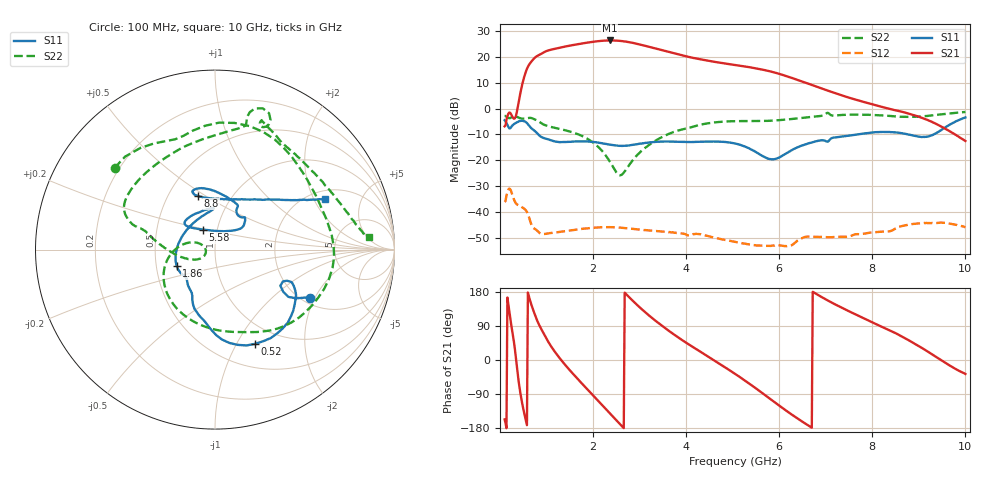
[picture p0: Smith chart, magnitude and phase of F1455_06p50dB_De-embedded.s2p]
! Integrated Device Technology
! Corporate Headquarters
! 6024 Silver Creek Valley Road
! San Jose, CA 95138  USA
! Phone:  1-408-284-8200
! Toll Free:  1-800-223-1366
! Webpage:  http://www.idt.com/
! Timing and RF Division
! 515 Groton Road, Suite 102
! Westford, MA 01886-6024
! Device:  F1455
! Description: 6-bit 0.5 dB Transmit Variable Gain Amplifier
! Frequency:  1400.0 -  2300.00 MHz
! Package:  6x6 mm Thin QFN Plastic Package: 28 pin
! State:  13
! Atten State:  6.5 dB
! Voltage:  +5.00 Volts
! Current:  217.677 mA
! Data:  The device was measured on a the F1455 evaluation board which has
!  individual transmission lines to the RF pins.  Data was collected
!  using a calibrated network analyzer.  The evaluation board was
!  de-embedded using a TRL calibration technique.
!  The reference plane is the edge of the package pin.
!  Pin  1 = CSb
!  Pin  2 = DATA
!  Pin  3 = CLK
!  Pin  4 = RSET
!  Pin  5 = GND
!  Pin  6 = RFIN  = Port 1
!  Pin  7 = GND
!  Pin  8 = NC
!  Pin  9 = NC
!  Pin 10 = NC
!  Pin 11 = NC
!  Pin 12 = NC
!  Pin 13 = NC
!  Pin 14 = /STBY
!  Pin 15 = GND
!  Pin 16 = RFOUT  = Port 2
!  Pin 17 = GND
!  Pin 18 = NC
!  Pin 19 = NC
!  Pin 20 = NC
!  Pin 21 = GND
!  Pin 22 = NC
!  Pin 23 = GND
!  Pin 24 = NC
!  Pin 25 = NC
!  Pin 26 = NC
!  Pin 27 = GND
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# GHz S dB R 50
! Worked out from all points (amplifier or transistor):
!   496 points, 100 MHz to 10 GHz, reference 50 ohm
!   highest |S21| = 26.4 dB at 2.36 GHz (marker M1)
!   |S21| within 3 dB of that: 1.234 GHz to 3.315 GHz (2.082 GHz wide, 91.5 % of centre)
!   unconditionally stable (mu >= 1): start of sweep to end of sweep
!   at 1.74 GHz: K = 5.08, MAG = 25.8 dB, |S12| = -46.6 dB
!   at 5.06 GHz: K = 17.46, MAG = 18.8 dB, |S12| = -51.6 dB
!   at 10 GHz: K = 57.77, MAG = -3.9 dB, |S12| = -45.9 dB
!   S11 on the Smith chart (normalised r, x): 100 MHz: 2.22, -1.84; 520 MHz: 0.77, -1.19; 1.86 GHz: 0.64, -0.12; 5.58 GHz: 0.85, +0.19; 8.8 GHz: 0.70, +0.46; 10 GHz: 2.35, +2.46
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0.1  -4.50 -26.8  -6.85 -156.8  -36.12 42.5  -2.84 140.9
0.38  -5.14 -38.1  0.23 -35.2  -37.23 -109.2  -3.30 55.9
0.52  -4.88 -67.0  12.22 -139.8  -38.71 -155.0  -3.92 24.3
0.7  -7.98 -98.9  18.76 136.9  -45.75 151.1  -3.78 -19.6
0.96  -11.48 -120.2  21.96 65.1  -48.50 123.1  -6.32 -72.2
1.14  -12.51 -130.8  23.00 28.5  -48.04 100.2  -7.27 -97.2
1.34  -12.94 -136.8  23.81 -3.8  -47.56 78.1  -8.10 -121.2
1.76  -12.63 -152.3  25.21 -61.9  -46.52 42.4  -10.54 -160.8
1.86  -12.68 -157.3  25.50 -74.9  -46.35 34.9  -11.47 -169.2
2.12  -13.18 -173.9  26.13 -108.8  -45.98 17.0  -14.96 170.4
2.36  -13.95 163.6  26.39 -140.5  -45.86 1.2  -20.45 158.7
2.54  -14.38 143.3  26.28 -164.2  -46.02 -10.0  -25.46 177.2
2.74  -14.27 121.6  25.84 170.1  -46.32 -20.9  -22.76 -149.3
3.06  -13.42 98.5  24.58 132.6  -46.90 -35.9  -16.09 -160.2
3.4  -12.80 92.0  22.98 98.0  -47.45 -49.4  -11.81 -178.7
4.1  -12.94 112.7  19.83 37.8  -48.83 -72.5  -7.24 164.1
5.06  -13.54 140.3  16.87 -37.3  -51.59 -107.9  -4.84 148.8
5.58  -17.71 121.7  15.33 -82.0  -52.95 -114.8  -4.79 128.5
6.7  -13.10 42.0  9.17 -178.6  -49.56 -144.7  -3.20 78.5
8.36  -9.04 109.4  -0.06 78.7  -47.49 163.0  -2.82 62.4
8.8  -10.08 107.5  -1.99 50.8  -44.84 147.9  -3.18 46.0
10  -3.41 24.9  -12.51 -36.9  -45.87 76.1  -1.30 4.6
